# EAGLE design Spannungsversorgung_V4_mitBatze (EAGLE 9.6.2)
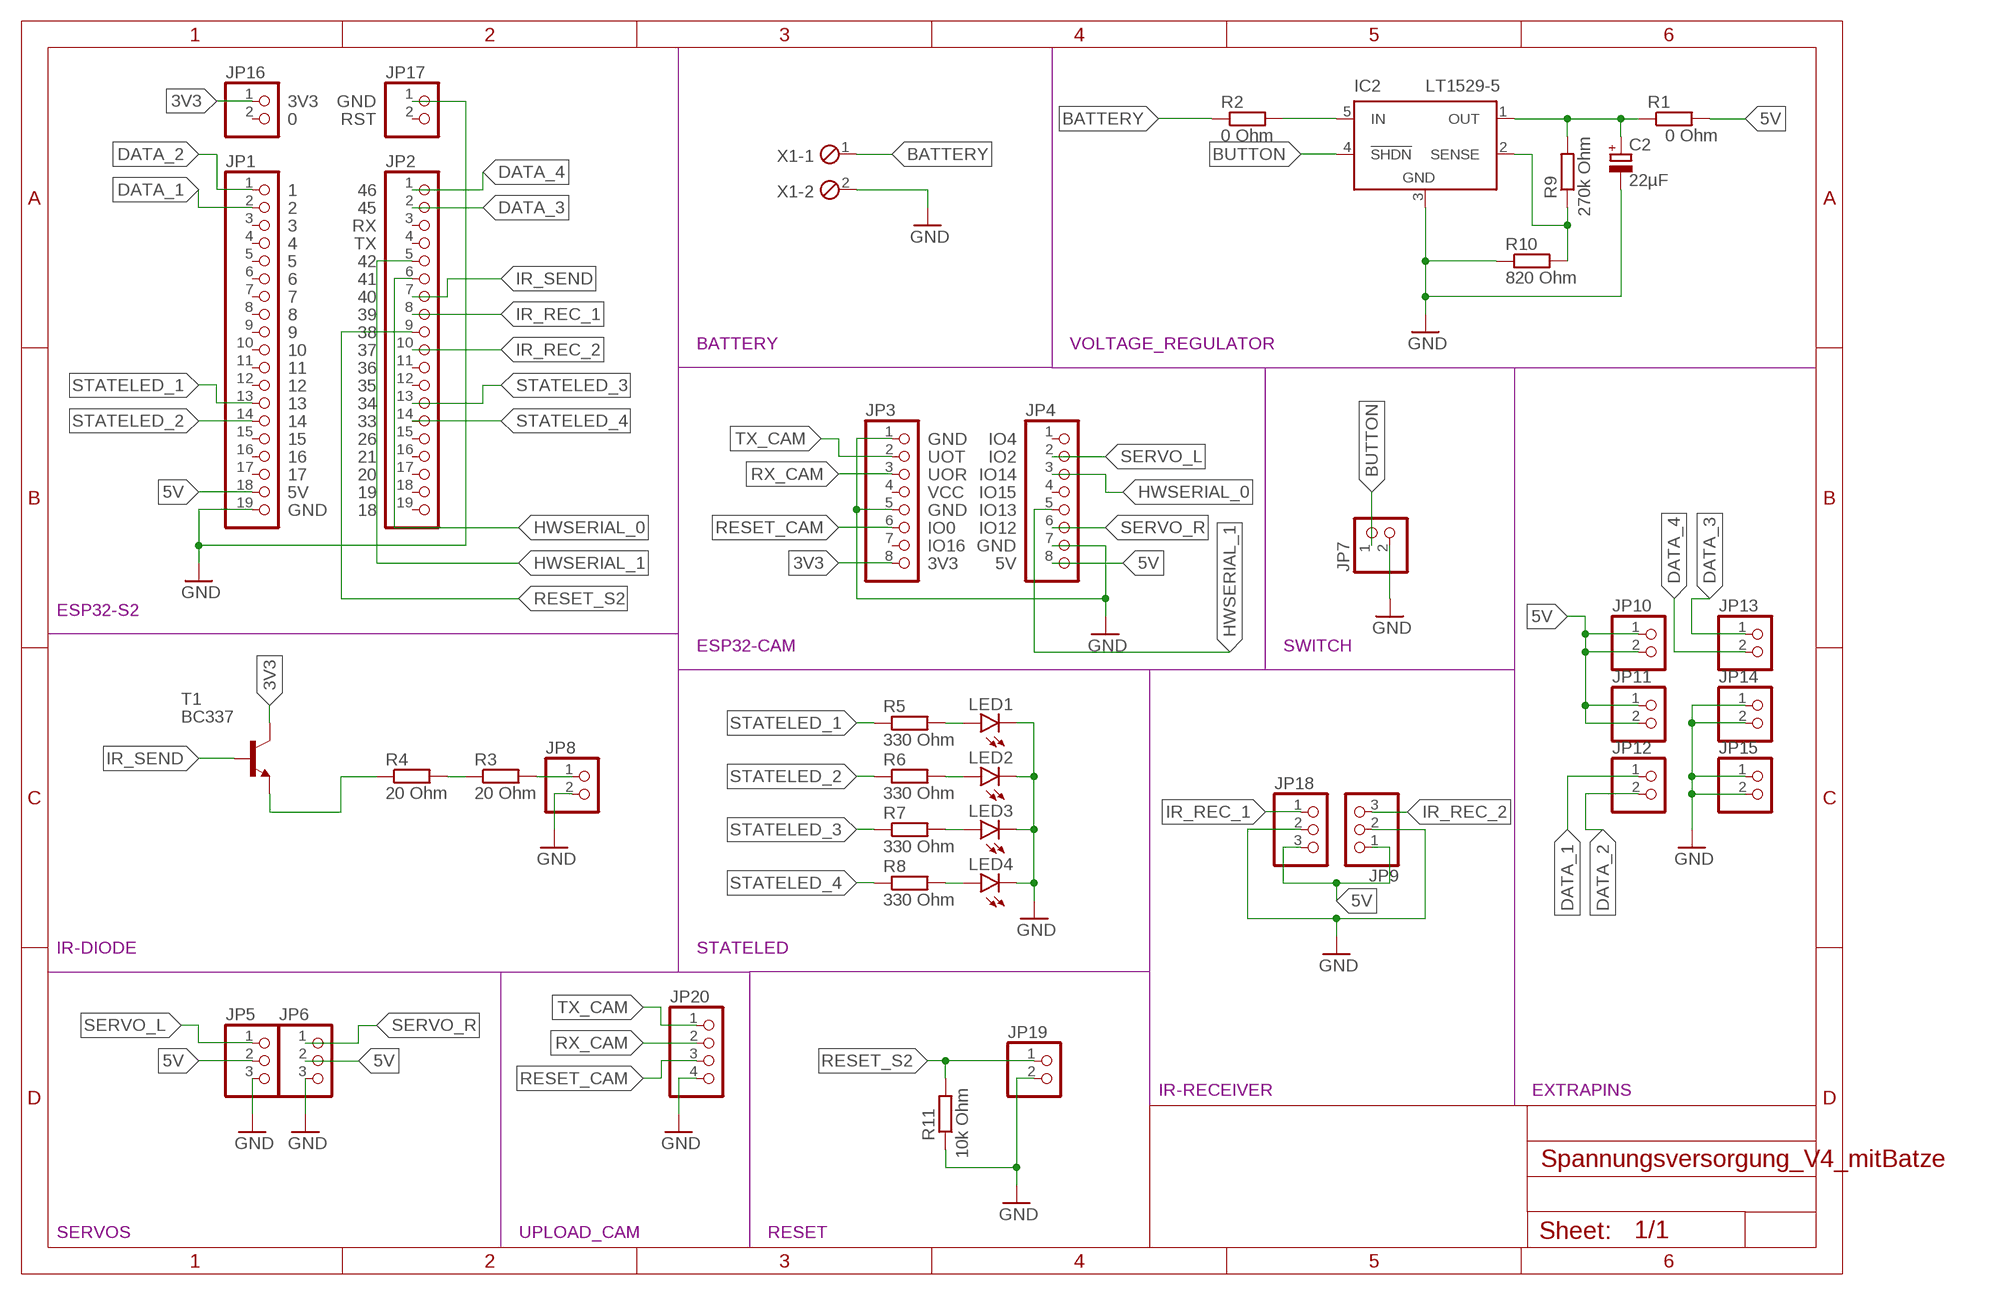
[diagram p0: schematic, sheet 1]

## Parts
C2  22µF  CPOL-EUE2.5-5  [E2,5-5]
IC2  LT1529-5  LT1529T  [TO220-5]
JP1  PINHD-1X19  [1X19]
JP2  PINHD-1X19  [1X19]
JP3  PINHD-1X8  [1X08]
JP4  PINHD-1X8  [1X08]
JP5  PINHD-1X3  [1X03]
JP6  PINHD-1X3  [1X03]
JP7  PINHD-1X2  [1X02]
JP8  PINHD-1X2  [1X02]
JP9  PINHD-1X3  [1X03]
JP10  PINHD-1X2  [1X02]
JP11  PINHD-1X2  [1X02]
JP12  PINHD-1X2  [1X02]
JP13  PINHD-1X2  [1X02]
JP14  PINHD-1X2  [1X02]
JP15  PINHD-1X2  [1X02]
JP16  PINHD-1X2  [1X02]
JP17  PINHD-1X2  [1X02]
JP18  PINHD-1X3  [1X03]
JP19  PINHD-1X2  [1X02]
JP20  PINHD-1X4  [1X04]
LED1  LED3MM  [LED3MM]
LED2  LED3MM  [LED3MM]
LED3  LED3MM  [LED3MM]
LED4  LED3MM  [LED3MM]
R1  0 Ohm  R-EU_R0805  [R0805]
R2  0 Ohm  R-EU_R0805  [R0805]
R3  20 Ohm  R-EU_0309/12  [0309/12]
R4  20 Ohm  R-EU_0309/12  [0309/12]
R5  330 Ohm  R-EU_R0805  [R0805]
R6  330 Ohm  R-EU_R0805  [R0805]
R7  330 Ohm  R-EU_R0805  [R0805]
R8  330 Ohm  R-EU_R0805  [R0805]
R9  270k Ohm  R-EU_0309/12  [0309/12]
R10  820 Ohm  R-EU_0309/12  [0309/12]
R11  10k Ohm  R-EU_0309/12  [0309/12]
T1  BC337  [TO92]
X1  MPT2  [2POL254]

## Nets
3V3: JP3.8 JP16.1 T1.3(C)
5V: JP1.18 JP4.8 JP5.2 JP6.2 JP9.1 JP10.1 JP10.2 JP11.1 JP11.2 JP18.3 R1.2
BATTERY: R2.1 X1.1
BUTTON: IC2.4(!SHDN) JP7.1
DATA_1: JP1.2 JP12.1
DATA_2: JP1.1 JP12.2
DATA_3: JP2.2 JP13.1
DATA_4: JP2.1 JP13.2
GND: C2.- IC2.3(GND) JP1.19 JP3.1 JP3.5 JP4.7 JP5.3 JP6.3 JP7.2 JP8.2 JP9.2 JP14.1 JP14.2 JP15.1 JP15.2 JP17.1 JP18.2 JP19.2 JP20.4 LED1.K(C) LED2.K(C) LED3.K(C) LED4.K(C) R10.1 R11.1 X1.2
HWSERIAL_0: JP2.6 JP4.3
HWSERIAL_1: JP2.5 JP4.5
IR_REC_1: JP2.8 JP18.1
IR_REC_2: JP2.10 JP9.3
IR_SEND: JP2.7 T1.2(B)
N$1: R3.1 R4.2
N$2: JP8.1 R3.2
N$3: IC2.5(IN) R2.2
N$5: LED1.A R5.2
N$6: LED2.A R6.2
N$7: LED3.A R7.2
N$8: LED4.A R8.2
N$11: R4.1 T1.1(E)
N$13: IC2.2(SENSE) R9.1 R10.2
N$14: C2.+ IC2.1(OUT) R1.1 R9.2
RESET_CAM: JP3.6 JP20.3
RESET_S2: JP2.9 JP19.1 R11.2
RX_CAM: JP3.3 JP20.2
SERVO_L: JP4.2 JP5.1
SERVO_R: JP4.6 JP6.1
STATELED_1: JP1.13 R5.1
STATELED_2: JP1.14 R6.1
STATELED_3: JP2.13 R7.1
STATELED_4: JP2.14 R8.1
TX_CAM: JP3.2 JP20.1
Unconnected: JP1.3 JP1.4 JP1.5 JP1.6 JP1.7 JP1.8 JP1.9 JP1.10 JP1.11 JP1.12 JP1.15 JP1.16 JP1.17 JP2.3 JP2.4 JP2.11 JP2.12 JP2.15 JP2.16 JP2.17 JP2.18 JP2.19 JP3.4 JP3.7 JP4.1 JP4.4 JP16.2 JP17.2

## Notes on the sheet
- 3V3 | GND
- 0 | RST
- 1 | 46
- 2 | 45
- 3 | RX
- 4 | TX
- 5 | 42
- 6 | 41
- 7 | 40
- 8 | 39
- 9 | 38
- BATTERY | VOLTAGE_REGULATOR
- 10 | 37
- 11 | 36
- 12 | 35
- 13 | 34
- 14 | 33
- 15 | 26 | GND | IO4
- 16 | 21 | UOT | IO2
- 17 | 20 | UOR | IO14
- 5V | 19 | VCC | IO15
- GND | 18 | GND | IO13
- IO0 | IO12
- IO16 | GND
- 3V3 | 5V
- ESP32-S2
- ESP32-CAM | SWITCH
- IR-DIODE | STATELED
- IR-RECEIVER | EXTRAPINS
- SERVOS | UPLOAD_CAM | RESET

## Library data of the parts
C2 = rcl:CPOL-EU: POLARIZED CAPACITOR, European symbol; SPICEPREFIX: C
IC2 = ltc1440_lt1529_ds1302:LT1529: LT1529 5 Volt LDO Regulator 5 Volt, 3 Ampere Low Dropout voltage regulator.
JP1 JP2 = pinhead:PINHD-1X19: PIN HEADER
JP3 JP4 = pinhead:PINHD-1X8: PIN HEADER
JP5 JP6 JP9 JP18 = pinhead:PINHD-1X3: PIN HEADER
JP7 JP8 JP10-JP17 JP19 = pinhead:PINHD-1X2: PIN HEADER
JP20 = pinhead:PINHD-1X4: PIN HEADER
LED1-LED4 = led:LED: LED
R1-R11 = rcl:R-EU_: RESISTOR, European symbol; SPICEPREFIX: R
T1 = transistor:BC337: NPN TRANSISTOR
X1 = con-phoenix-254:MPT2: PHOENIX CONNECTOR; OC_FARNELL: unknown; OC_NEWARK: unknown

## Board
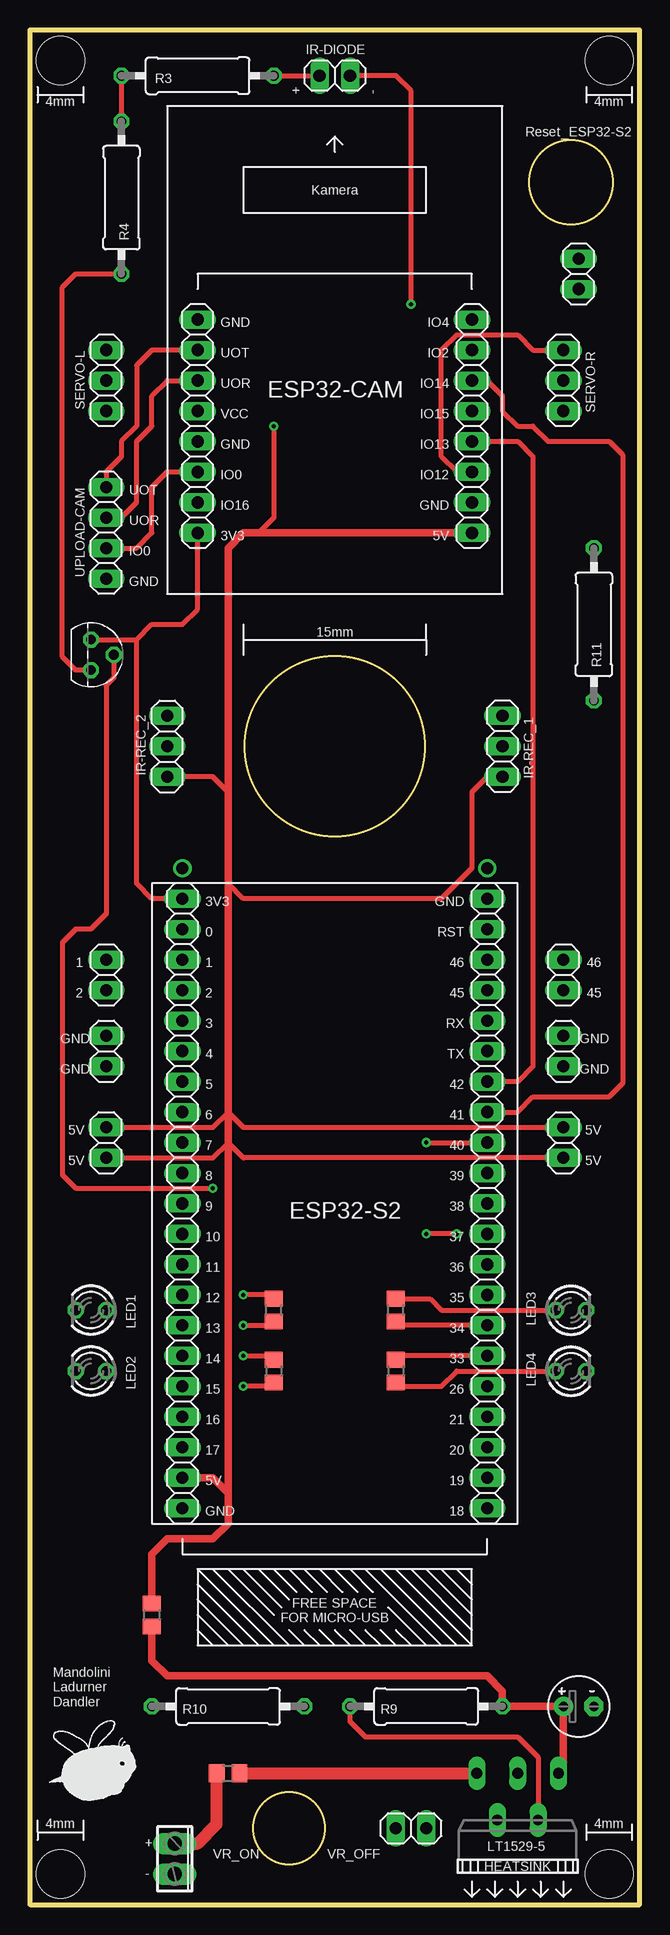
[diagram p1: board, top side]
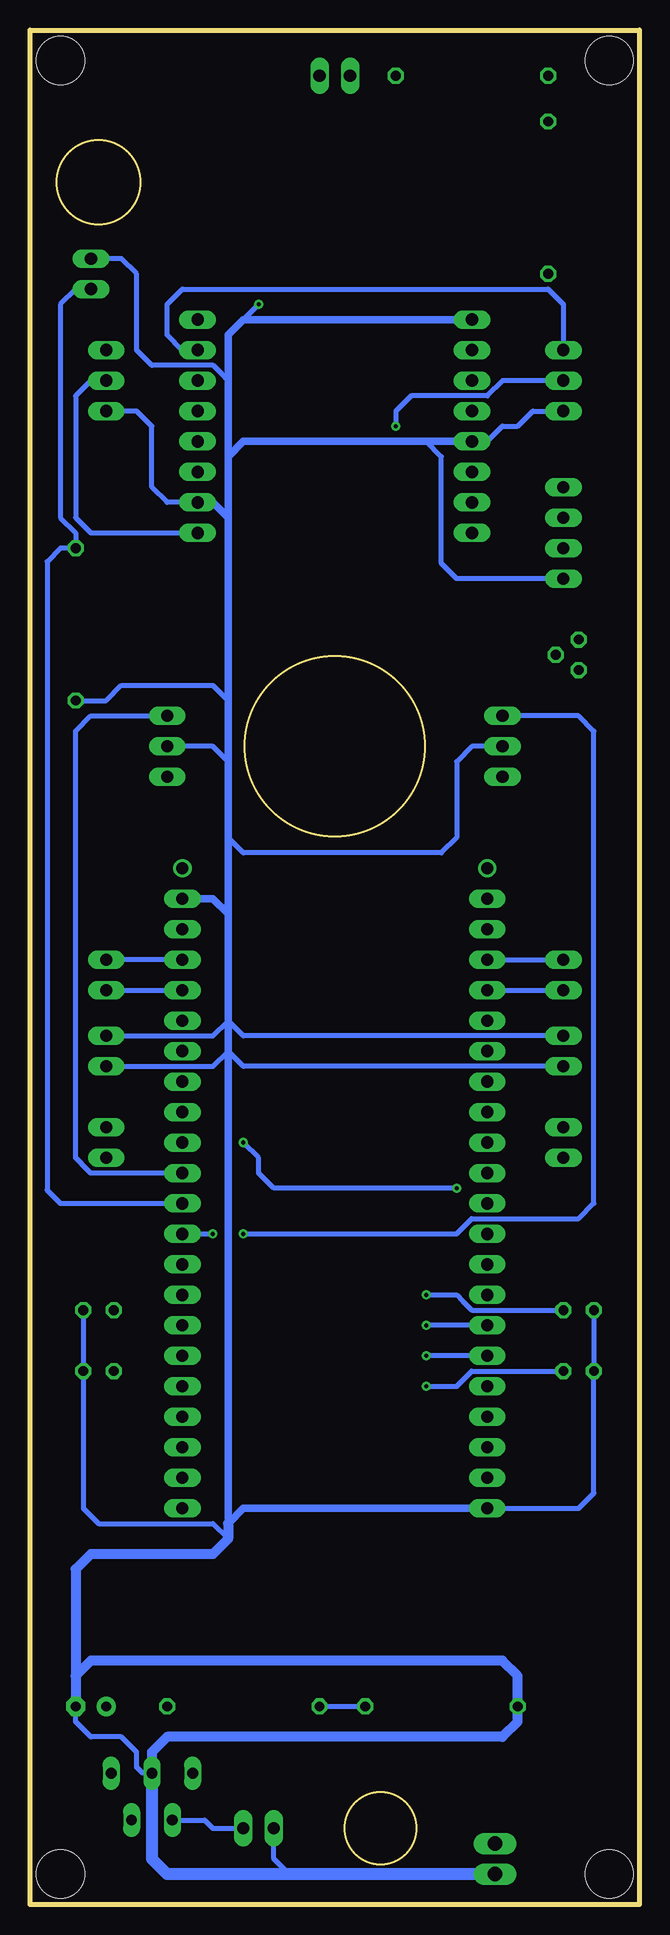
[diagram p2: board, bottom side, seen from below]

Size 50.8 x 156.21 mm. Coordinates in mm from the lower left corner, seen from the top.
Outline: 0,0 50.8,0 50.8,156.21 0,156.21 0,0
Copper layers (1*16): Top 0.035mm / dielectric 1.5mm / Bottom 0.035mm
Design rules "default *": minimum track width 6mil, minimum drill 0.35mm, track to track 12mil, track to pad 12mil, pad to pad 12mil, via to via 12mil, smd to smd 12mil, copper to edge 40mil, drill to drill 12mil, minimum pad ring 10mil, minimum via ring 8mil, stop-mask expansion 4mil, vias tented up to drill 0mil, thermal gap 10mil
Holes 4 mm at 2.54,153.67 48.26,153.67 48.26,2.54 2.54,2.54
Milling: area 17.9,89 to 32.9,104; area 18.6,3.4 to 24.6,9.3; area 41.6,140 to 48.6,147

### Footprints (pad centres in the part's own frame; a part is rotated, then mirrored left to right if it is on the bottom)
E2,5-5 = drill 0.813 pad 1.6: + -1.27,0 | drill 0.813 pad 1.6 octagon: - 1.27,0
TO220-5 = drill 0.9 long: 1 -3.4,-8.4; 2 -1.7,-4.5; 3 0,-8.4; 4 1.7,-4.5; 5 3.4,-8.4
1X19 = drill 1.016 long: 1 -22.86,0; 2 -20.32,0; 3 -17.78,0; 4 -15.24,0; 5 -12.7,0; 6 -10.16,0; 7 -7.62,0; 8 -5.08,0; 9 -2.54,0; 10 0,0; 11 2.54,0; 12 5.08,0; 13 7.62,0; 14 10.16,0; 15 12.7,0; 16 15.24,0; 17 17.78,0; 18 20.32,0; 19 22.86,0
1X08 = drill 1.016 long: 1 -8.89,0; 2 -6.35,0; 3 -3.81,0; 4 -1.27,0; 5 1.27,0; 6 3.81,0; 7 6.35,0; 8 8.89,0
1X03 = drill 1.016 long: 1 -2.54,0; 2 0,0; 3 2.54,0
1X02 = drill 1.016 long: 1 -1.27,0; 2 1.27,0
1X04 = drill 1.016 long: 1 -3.81,0; 2 -1.27,0; 3 1.27,0; 4 3.81,0
LED3MM = drill 0.813 octagon: A -1.27,0; K 1.27,0
R0805 = smd 1.3 x 1.5: 1 -0.95,0; 2 0.95,0
0309/12 = drill 0.813 octagon: 1 -6.35,0; 2 6.35,0
TO92 = drill 0.813 octagon: 1 1.27,0; 2 0,1.905; 3 -1.27,0
2POL254 = drill 1.2 long: 1 -1.27,0; 2 1.27,0

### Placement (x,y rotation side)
C2  45.72,16.51 0 top
IC2  40.64,2.54 180 top
JP1  12.7,55.88 270 top
JP2  38.1,55.88 270 top
JP3  13.97,123.19 270 top
JP4  36.83,123.19 270 top
JP5  6.35,127 270 top
JP6  44.45,127 270 top
JP7  31.75,6.35 180 top
JP8  25.4,152.4 0 top
JP9  11.43,96.52 90 top
JP10  6.35,63.5 90 top
JP11  44.45,63.5 90 top
JP12  6.35,77.47 90 top
JP13  44.45,77.47 90 top
JP14  6.35,71.12 90 top
JP15  44.45,71.12 90 top
JP16  12.7,82.55 270 top
JP17  38.1,82.55 270 top
JP18  39.37,96.52 270 top
JP19  45.72,135.89 90 top
JP20  6.35,114.3 270 top
LED1  5.08,49.53 180 top
LED2  5.08,44.45 180 top
LED3  45.09,49.53 0 top
LED4  45.09,44.45 0 top
R1  10.16,24.13 90 top
R2  16.51,10.93 0 top
R3  13.97,152.4 0 top
R4  7.62,142.24 90 top
R5  20.32,49.53 90 top
R6  20.32,44.45 270 top
R7  30.48,49.53 90 top
R8  30.48,44.45 270 top
R9  33.02,16.51 0 top
R10  16.51,16.51 0 top
R11  46.99,106.68 90 top
T1  5.08,104.14 270 top
X1  12.06,3.81 270 top

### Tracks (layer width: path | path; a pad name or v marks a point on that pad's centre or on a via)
3V3
  Top 0.406: 8.89,105.41 8.89,85.09 10.16,83.82 JP16.1 | 8.89,105.41 10.16,106.68 12.7,106.68 13.97,107.95 JP3.8 | T1.3 8.89,105.41
5V  (via drill 0.35)
  Top 0.406: JP10.2 15.24,64.77 16.51,66.04 17.78,64.77 JP11.2 | JP10.1 15.24,62.23 16.51,63.5 17.78,62.23 JP11.1 | 16.51,92.71 15.24,93.98 JP9.1 | 16.51,85.09 17.78,83.82 34.29,83.82 36.83,86.36 36.83,92.71 38.1,93.98 JP18.3 | v20.32,123.19 20.32,115.57 19.05,114.3
  Top 0.61: R1.2 10.16,29.21 11.43,30.48 15.24,30.48 16.51,31.75 16.51,34.29 | JP4.8 19.05,114.3 17.78,114.3 16.51,113.03 16.51,92.71 16.51,85.09 16.51,66.04 16.51,63.5 16.51,34.29 | 16.51,34.29 15.24,35.56 JP1.18
  Bottom 0.406: JP6.2 45.72,127 46.99,125.73 46.99,115.57 45.72,114.3 JP4.8 | JP5.2 11.41,127 12.68,125.73 19.05,125.73 20.32,124.46 v20.32,123.19
BATTERY
  Top 1.016: X1.1 13.97,5.08 15.56,6.67 R2.1
BUTTON
  Bottom 0.406: IC2.4 36.25,7.04 35.56,6.35 JP7.1
DATA_1
  Bottom 0.406: JP1.2 JP12.1
DATA_2
  Bottom 0.406: JP1.1 JP12.2
DATA_3
  Bottom 0.406: JP13.1 JP2.2
DATA_4
  Bottom 0.406: JP2.1 JP13.2
GND  (via drill 0.35)
  Top 0.406: v31.75,133.35 31.75,151.13 30.48,152.4 JP8.2
  Bottom 0.406: 29.21,2.54 30.48,3.81 JP7.2 | IC2.3 41.42,10.94 41.91,11.43 41.91,12.7 43.18,13.97 45.72,13.97 46.99,15.24 C2.- | JP14.2 33.02,72.39 34.29,73.66 35.56,72.39 JP15.2 | JP14.1 33.02,69.85 34.29,71.12 35.56,69.85 JP15.1 | 34.29,95.25 35.56,96.52 JP18.2 | JP9.2 13.97,96.52 15.24,95.25 15.24,88.9 16.51,87.63 33.02,87.63 34.29,88.9 | LED1.K LED2.K 3.81,34.29 5.08,33.02 JP1.19 | LED3.K LED4.K 46.36,33.02 45.09,31.75 35.56,31.75 34.29,30.48 | JP4.7 39.37,116.84 40.64,118.11 40.64,123.19 41.91,124.46 JP6.3 | JP3.5 12.7,121.92 11.43,123.19 10.16,123.19 8.89,124.46 JP5.3 | JP20.4 15.24,110.49 16.51,111.76 16.51,120.65 17.78,121.92 | 33.02,132.08 v31.75,133.35 | 34.29,127 34.8,127.51 34.8,127.53 35.54,128.27 40.64,128.27 41.91,129.54 41.91,135.89 43.18,137.16 JP19.2 | R11.1 44.45,100.33 43.18,101.6 35.56,101.6 34.29,100.33
  Bottom 0.61: JP4.7 35.56,116.84 34.29,115.57 | 34.29,115.57 34.29,100.33 34.29,95.25 34.29,88.9 34.29,82.55 | 34.29,82.55 34.29,73.66 34.29,71.12 34.29,31.75 33.02,33.02 JP1.19 | JP17.1 35.56,83.82 34.29,82.55 | 34.29,120.65 34.29,127 34.29,130.81 33.02,132.08 JP3.1 | 34.29,120.65 34.29,115.57 | JP3.5 17.78,121.92 33.02,121.92 34.29,120.65
  Bottom 0.813: IC2.3 40.64,12.7 39.37,13.97 11.43,13.97 10.16,15.24 R10.1 10.16,19.05 11.43,20.32 45.72,20.32 46.99,19.05 | 34.29,31.75 34.29,30.48 35.56,29.21 45.72,29.21 46.99,27.94 46.99,19.05 | 46.99,19.05 C2.-
  Bottom 1.016: IC2.3 40.64,3.81 39.37,2.54 29.21,2.54 X1.2
HWSERIAL_0
  Top 0.406: JP2.6 40.64,66.04 41.91,67.31 48.26,67.31 49.38,68.43 49.38,120.8 48.26,121.92 43.18,121.92 41.91,123.19 40.64,123.19 39.37,124.46 39.37,125.73 38.1,127 JP4.3
HWSERIAL_1
  Top 0.406: JP4.5 40.64,121.92 41.91,120.65 41.91,69.85 40.64,68.58 JP2.5
IR_REC_1
  Bottom 0.406: JP18.1 45.72,99.06 46.99,97.79 46.99,62.23 46.48,61.72 46.48,61.7 45.74,60.96 JP2.8
IR_REC_2  (via drill 0.35)
  Top 0.406: v35.56,55.88 v33.02,55.88
  Bottom 0.406: JP2.10 v35.56,55.88 | v33.02,55.88 15.24,55.88 14.73,56.39 14.73,56.41 13.99,57.15 5.08,57.15 3.81,58.42 3.81,97.79 5.08,99.06 JP9.3
IR_SEND  (via drill 0.35)
  Top 0.406: T1.2 6.98,102.23 6.35,101.6 6.35,82.55 5.08,81.28 3.81,81.28 2.69,80.16 2.69,60.81 3.81,59.69 v15.24,59.69 | v33.02,63.5 JP2.7
  Bottom 0.406: v33.02,63.5 31.75,62.23 31.75,60.96 30.48,59.69 v15.24,59.69
N$1
  Top 0.406: R3.1 R4.2
N$2
  Top 0.406: R3.2 JP8.1
N$3
  Top 1.016: R2.2 IC2.5
N$5  (via drill 0.35)
  Top 0.406: R5.2 20,50.8 v17.78,50.8
  Bottom 0.406: v17.78,50.8 15.24,50.8 14.73,50.29 14.73,50.27 13.99,49.53 LED1.A
N$6  (via drill 0.35)
  Top 0.406: R6.2 20,43.18 v17.78,43.18
  Bottom 0.406: v17.78,43.18 15.24,43.18 14.73,43.69 14.73,43.71 13.99,44.45 LED2.A
N$7
  Top 0.406: R7.2 33.34,50.48 34.29,49.53 LED3.A
N$8
  Top 0.406: R8.2 30.8,43.18 34.29,43.18 35.56,44.45 LED4.A
N$9  (via drill 1.02)
  other vias: 38.1,86.36
N$10  (via drill 1.02)
  other vias: 12.7,86.36
N$11
  Top 0.406: T1.1 3.81,102.87 2.69,103.99 2.69,134.77 3.81,135.89 R4.1
N$13
  Top 0.406: R9.1 26.67,15.24 27.94,13.97 40.64,13.97 42.34,12.27 IC2.2
  Bottom 0.406: R9.1 R10.2
N$14
  Top 0.61: IC2.1 44.45,11.35 C2.+ R9.2 39.37,17.78 38.1,19.05 11.43,19.05 10.16,20.32 R1.1
RESET_CAM
  Top 0.406: JP3.6 11.43,119.38 10.16,118.11 10.16,114.3 8.89,113.03 JP20.3
RESET_S2
  Bottom 0.406: JP19.1 46.99,134.62 48.26,133.35 48.26,115.57 46.99,114.3 R11.2 48.26,113.03 49.38,111.91 49.38,59.54 48.26,58.42 JP2.9
RX_CAM
  Top 0.406: JP20.2 7.62,115.57 8.89,116.84 8.89,121.92 10.16,123.19 10.16,125.73 11.43,127 JP3.3
SERVO_L
  Bottom 0.406: JP4.2 38.1,129.54 39.37,130.81 39.37,133.35 38.1,134.62 7.62,134.62 6.35,133.35 JP5.1
SERVO_R
  Top 0.406: JP4.6 35.56,119.38 34.29,120.65 34.29,129.56 35.54,130.81 40.64,130.81 41.91,129.54 JP6.1
STATELED_1  (via drill 0.35)
  Top 0.406: v17.78,48.26 20,48.26 R5.1
  Bottom 0.406: JP1.13 v17.78,48.26
STATELED_2  (via drill 0.35)
  Top 0.406: v17.78,45.72 20,45.72 R6.1
  Bottom 0.406: JP1.14 v17.78,45.72
STATELED_3
  Top 0.406: R7.1 30.8,48.26 JP2.13
STATELED_4
  Top 0.406: R8.1 30.8,45.72 JP2.14
TX_CAM
  Top 0.406: JP3.2 10.16,129.54 8.89,128.27 8.89,123.19 7.62,121.92 7.62,120.65 6.35,119.38 JP20.1

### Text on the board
tPlace: ESP32-CAM | ESP32-S2
tNames: IR-DIODE | + | - | 4mm | 4mm | Reset_ESP32-S2 | Kamera | GND | IO4 | UOT | IO2 | UOR | IO14 | SERVO-L | VCC | IO15 | SERVO-R | GND | IO13 | IO0 | IO12 | UOT | IO16 | GND | UOR | 3V3 | 5V | IO0 | UPLOAD-CAM | GND | 15mm | IR-REC_1 | IR-REC_2 | 3V3 | GND | 0 | RST | 1 | 1 | 46 | 46 | 2 | 2 | 45 | 45 | 3 | RX | GND | GND | 4 | TX | GND | GND | 5 | 42 | 6 | 41 | 5V | 5V | 7 | 40 | 5V | 5V | 8 | 39 | 9 | 38 | 10 | 37 | 11 | 36 | 12 | 35 | 13 | 34 | 14 | 33 | 15 | 26 | 16 | 21 | 17 | 20 | 5V | 19 | GND | 18 | FREE SPACE / FOR MICRO-USB | Mandolini / Ladurner / Dandler | 4mm | 4mm | + | VR_ON | VR_OFF | HEATSINK | -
